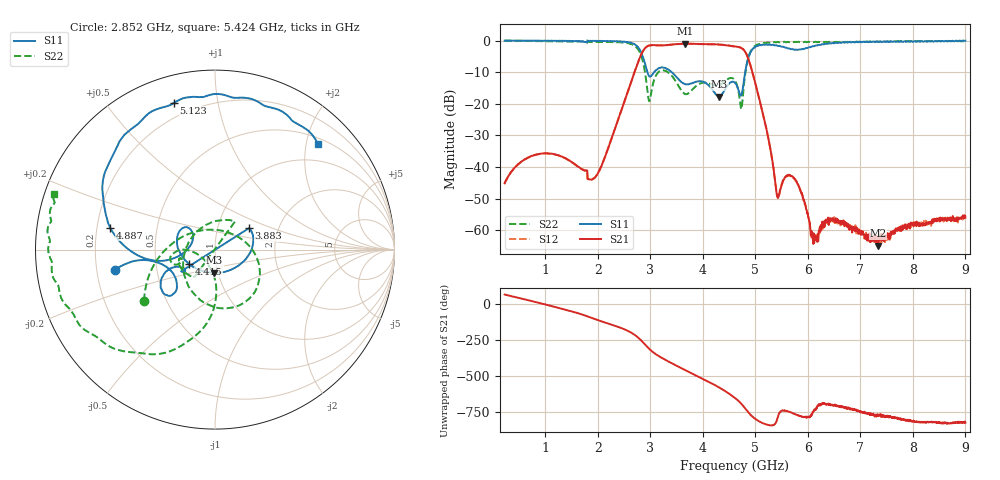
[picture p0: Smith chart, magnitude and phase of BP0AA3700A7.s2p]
!Agilent Technologies,E8358A,US41080443,A.07.50.56
!Agilent E8358A: A.07.50.56
!Date: Wednesday, May 23, 2018 14:50:04
!Correction: S11(Full 2 Port(1,2))
!S21(Full 2 Port(1,2))
!S12(Full 2 Port(1,2))
!S22(Full 2 Port(1,2))
!S2P File: Measurements: S11, S21, S12, S22:
# Hz S  dB  R 50
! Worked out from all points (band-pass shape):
!   1601 points, 225 MHz to 9 GHz, reference 50 ohm
!   highest |S21| = -0.99 dB at 3.664 GHz (marker M1); lowest = -64.8 dB at 7.338 GHz (marker M2)
!   |S21| within 3 dB of the highest: 2.84 GHz to 4.821 GHz (1.981 GHz wide, 51.7 % of centre)
!   lowest |S11| = -17.8 dB at 4.311 GHz (marker M3), VSWR 1.30, Z = 47.9 - j12.6 ohm
!   |S11| at or under -10 dB: 2.943 GHz to 3.074 GHz (130.7 MHz wide, 4.34 % of centre); 3.407 GHz to 4.807 GHz (1.4 GHz wide, 34.1 % of centre)
!   |S22| runs from -21.7 to 0.0 dB; largest |S21 - S12| = 0.0068
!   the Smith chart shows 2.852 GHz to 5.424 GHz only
!   S11 on the Smith chart (normalised r, x): 2.852 GHz: 0.28, -0.09; 3.883 GHz: 1.42, +0.36; 4.415 GHz: 0.74, -0.12; 4.887 GHz: 0.25, +0.10; 5.123 GHz: 0.13, +0.75; 5.424 GHz: 0.61, +2.23
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2.25e8  -0.02 -7.7  -45.15 68.8  -45.16 69.2  -0.05 -32.2
6.472969e8  -0.07 -22.8  -37.23 31.9  -37.24 31.7  -0.14 -92.4
1.086047e9  -0.11 -41.2  -35.75 -8.5  -35.75 -8.1  -0.25 -155.6
1.689328e9  -0.33 -79.6  -40.63 -67.9  -40.61 -68.4  -0.26 120.7
2.281641e9  -0.23 -95.2  -30.02 -142.9  -30.05 -143.3  -0.53 1.6
2.665547e9  -0.95 -134.8  -11.64 158.0  -11.66 157.7  -1.35 -72.6
2.852016e9  -4.88 -168.5  -3.61 100.1  -3.63 99.9  -6.25 -144.3
3.153656e9  -8.76 -134.9  -1.51 2.9  -1.57 3.0  -10.00 -42.6
3.663703e9  -13.81 -149.3  -0.99 -96.3  -1.04 -96.5  -16.93 140.6
3.883078e9  -12.98 32.2  -1.06 -136.0  -1.11 -136.0  -14.23 -126.8
4.310859e9  -17.77 -92.0  -1.26 142.9  -1.28 142.8  -14.08 -161.8
4.415062e9  -15.65 -150.8  -1.44 120.1  -1.47 120.1  -12.92 -158.5
4.6125e9  -13.35 145.9  -1.86 70.8  -1.90 70.8  -12.72 -175.0
4.733156e9  -17.29 167.6  -2.35 30.0  -2.39 29.9  -21.70 -135.6
4.886719e9  -4.48 168.2  -6.74 -38.2  -6.81 -38.0  -4.37 -112.5
5.122547e9  -1.42 105.6  -21.68 -101.5  -21.73 -102.1  -0.96 -166.2
5.424188e9  -1.69 45.8  -49.64 -65.6  -48.90 -67.7  -0.44 161.0
5.808094e9  -2.95 -69.1  -45.38 -49.7  -45.49 -49.8  -0.42 129.9
6.076828e9  -1.86 -149.5  -61.04 -43.9  -60.54 -40.0  -0.40 109.3
7.338234e9  -0.43 97.5  -64.81 -52.1  -63.57 -39.3  -0.35 23.3
7.541156e9  -0.46 89.2  -61.12 -63.4  -61.13 -64.6  -0.34 13.6
9e9  -0.07 51.8  -56.01 -101.8  -55.78 -98.9  -0.24 -21.0
